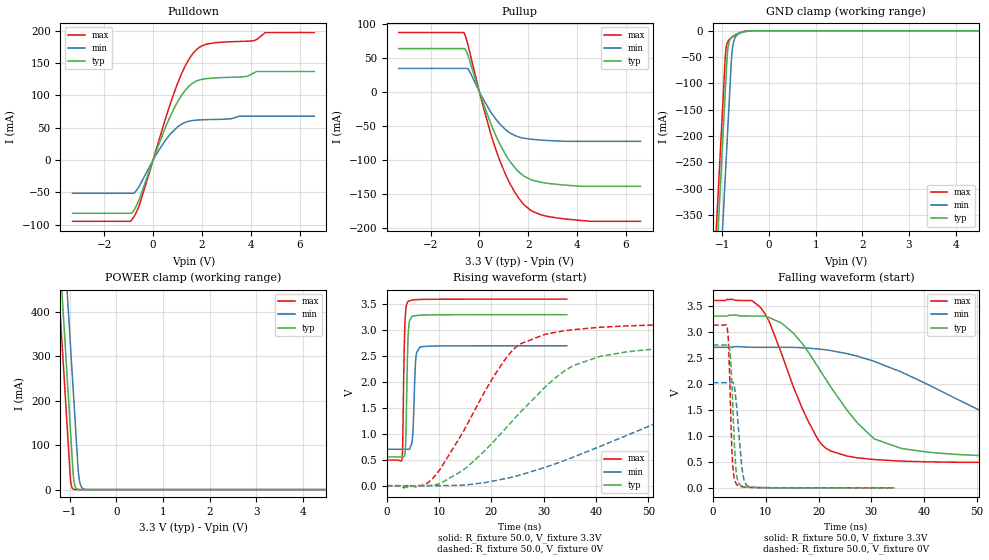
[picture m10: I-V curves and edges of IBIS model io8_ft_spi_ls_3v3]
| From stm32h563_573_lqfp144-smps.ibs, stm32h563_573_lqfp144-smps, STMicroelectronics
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[Model]   io8_ft_spi_ls_3v3
Model_type I/O
Polarity   Non-Inverting
Enable   Active-Low
| CAP_THRESHOLD on pad IOFT is "UDTCAPC" :
| Rising=20.0% of vddiom   Falling=80.0% of vddiom
| C_comp min and max val. don't necessarily correlate with the min and max pvt
| but are the smallest and greatest pad capacitance found.
| var   typ   min   max
C_comp   5.03667pF  4.97381pF  5.04450pF
|C_comp_pullup   3.26860pF  3.10795pF  3.04360pF
|C_comp_pulldown   1.76807pF  1.86586pF  2.00090pF
Vinl = 810.0mV
Vinh = 2.52V
Vmeas = 1.65V   | Reference voltage for timing measurements
Cref  = 50.0pF   | Timing specification test load capacitance value
Rref  = 100.0MOhm   | Timing specification test load resistance value
Vref  = 1.65V   | Timing specification test load voltage
[Model Spec]
| TIME_THRESHOLD on pin ZIV11 is "CMOS" :
| Rising=40.0% of vdd   Falling=60.0% of vdd
Vinl 1.29880V 1.07480V 1.40680V
Vinh 1.77520V 1.49320V 1.89720V
| variable   typ   min   max
[Temperature Range] 25.0 125.0 -40.0
| variable   typ   min   max
[Voltage Range] 3.3V 2.7V 3.6V
| variable   typ   min   max
[POWER Clamp Reference] 3.3V 2.7V 3.6V
| variable   typ   min   max
[GND Clamp Reference] 0V 0V 0V
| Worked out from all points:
|   slope of the pulldown table from 0 to 0.495 V, typ, clamps not added: 10 ohm
|   slope of the pullup table from 0 to 0.495 V, typ, clamps not added: 10 ohm
|   GND clamp passes 1 mA (typ) near -0.52 V on its own axis
|   POWER clamp passes 1 mA (typ) near -0.84 V on its own axis
|   rising waveform, R_fixture 50.0, V_fixture 3.3V: 20-80 % time 340ps typ, 425ps min, 327ps max; typ from 0.556 V to 3.3 V
|   falling waveform, R_fixture 50.0, V_fixture 3.3V: 20-80 % time 11.8ns typ, 26.7ns min, 7.44ns max; typ from 3.3 V to 0.556 V
|   rising waveform, R_fixture 50.0, V_fixture 0V: 20-80 % time 16.3ns typ, 32ns min, 11ns max; typ from 0 V to 2.74 V
|   falling waveform, R_fixture 50.0, V_fixture 0V: 20-80 % time 727ps typ, 1.05ns min, 588ps max; typ from 2.74 V to 0 V
[POWER Clamp]
-3.3V     4.068A     4.259A     3.957A
-1.25V    582.8mA    774.2mA    471.5mA
-1.13V    378.8mA    570.2mA    267.5mA
-1.09V    310.8mA    502.2mA    199.5mA
-1.02V    191.8mA    383.2mA    80.53mA
-990mV    140.8mA    332.2mA    29.53mA
-920mV    26.3mA     213.2mA    906uA
-880mV    5.543mA    145.2mA    123.7uA
-810mV    363.5uA    33.6mA     3.798uA
-770mV    76.62uA    10.47mA    519.4nA
-690mV    3.409uA    1.017mA    10.47nA
6.6V      0A         0A         0A
[GND Clamp]
-3.3V     -4.131A    -4.293A    -4.064A
-1.25V    -646.2mA   -808mA     -579.5mA
-940mV    -119.2mA   -281mA     -52.48mA
-920mV    -85.23mA   -247mA     -32.7mA
-900mV    -51.91mA   -213mA     -24.27mA
-870mV    -26.87mA   -162mA     -18.7mA
-810mV    -13.22mA   -60.41mA   -13.31mA
-790mV    -11.41mA   -38.37mA   -11.93mA
-740mV    -8.18mA    -15.37mA   -8.882mA
-660mV    -4.605mA   -6.274mA   -4.919mA
-320mV    -10.56uA   -77.76uA   -2.038uA
6.6V      9.514nA    1.879uA    704.5pA
| variable   typ   min   max
[Pullup Reference] 3.3V 2.7V 3.6V
| variable   typ   min   max
[Pulldown Reference] 0V 0V 0V
[Pullup]
-3.3V     63.89mA    34.71mA    87.52mA
-630mV    63.89mA    34.71mA    86.85mA
-430mV    49.62mA    32.06mA    63.53mA
120mV     -12.96mA   -8.365mA   -16.99mA
470mV     -47.29mA   -29.8mA    -62.21mA
800mV     -74.32mA   -45.73mA   -97.77mA
1.14V     -96.49mA   -57.59mA   -127.1mA
1.48V     -113mA     -64.78mA   -149.7mA
2.08V     -128.9mA   -69.61mA   -174.1mA
2.7V      -134.3mA   -71.45mA   -182.9mA
3.6V      -137.7mA   -72.9mA    -187.7mA
6.6V      -139.3mA   -72.9mA    -190.8mA
[Pulldown]
-3.3V     -82.43mA   -51.49mA   -94.82mA
-860mV    -81.66mA   -51.49mA   -91.78mA
-560mV    -60.16mA   -40.13mA   -69.41mA
120mV     12.61mA    7.999mA    15.37mA
800mV     75.3mA     43.94mA    97.52mA
1.33V     108.3mA    58.37mA    146.5mA
1.84V     123.1mA    61.83mA    172.7mA
2.51V     126.9mA    62.69mA    181.3mA
3.84V     129.3mA    67.77mA    183.7mA
4.13V     134.7mA    67.77mA    184.6mA
4.59V     136.9mA    67.77mA    197.1mA
6.6V      136.9mA    67.77mA    197.1mA
[Ramp]
dV/dt_r 1.64628V/16.22065ns 1.21218V/31.72839ns 1.87635V/10.80188ns
dV/dt_f 1.64665V/11.56808ns 1.19679V/26.48811ns 1.86387V/7.29972ns
R_load = 50.0
| Removed startup time: 0s 0s 0s  .
| Removed end time: 34.4ns.
[Rising Waveform]
R_fixture   = 50.0
V_fixture   = 3.3V
V_fixture_min = 2.7V
V_fixture_max = 3.6V
0s        555.6mV    703.3mV    493.6mV
2.9ns     555.7mV    703.3mV    509.6mV
3.05ns    553.1mV    703.3mV    815.2mV
3.4ns     581.7mV    703.4mV    2.898V
3.6ns     776.2mV    703.4mV    3.348V
4.1ns     2.914V     701mV      3.555V
4.85ns    3.266V     855.2mV    3.581V
5.55ns    3.282V     2.443V     3.589V
6.35ns    3.29V      2.676V     3.593V
34.4ns    3.3V       2.699V     3.6V
| Removed startup time: 0s 0s 0s  .
| Removed end time: 249.4ns.
[Falling Waveform]
R_fixture   = 50.0
V_fixture   = 3.3V
V_fixture_min = 2.7V
V_fixture_max = 3.6V
0s        3.3V       2.7V       3.6V
8.8ns     3.299V     2.7V       3.486V
15.25ns   2.97V      2.699V     1.934V
20.05ns   2.296V     2.667V     907.7mV
27.35ns   1.248V     2.53V      578mV
30.55ns   940.7mV    2.43V      543.7mV
40.75ns   685.5mV    1.984V     499.6mV
58.85ns   594.3mV    1.148V     488.3mV
76.35ns   570.4mV    888.9mV    490.3mV
249.4ns   555.6mV    705.3mV    493.6mV
| Removed startup time: 0s 0s 0s  .
| Removed end time: 249.4ns.
[Rising Waveform]
R_fixture   = 50.0
V_fixture   = 0V
V_fixture_min = 0V
V_fixture_max = 0V
0s        103.7nV    446.5nV    93.93nV
7.9ns     1.334mV    -337.5uV   59.97mV
14.5ns    293.5mV    10.02mV    1.02V
20.4ns    850.3mV    90.42mV    2.102V
24.6ns    1.316V     182.1mV    2.667V
35.6ns    2.315V     549.1mV    3.01V
45.8ns    2.581V     968.6mV    3.083V
61.1ns    2.69V      1.549V     3.114V
81.5ns    2.729V     1.872V     3.124V
249.4ns   2.744V     2.02V      3.127V
| Removed startup time: 0s 0s 0s  .
| Removed end time: 34.35ns.
[Falling Waveform]
R_fixture   = 50.0
V_fixture   = 0V
V_fixture_min = 0V
V_fixture_max = 0V
0s        2.744V     2.021V     3.127V
2.7ns     2.747V     2.021V     3.061V
2.95ns    2.742V     2.021V     2.734V
3.25ns    2.552V     2.021V     1.785V
3.7ns     1.715V     2.03V      476mV
4.2ns     555.7mV    1.83V      118.3mV
4.6ns     171.9mV    1.421V     54.6mV
5.7ns     26.13mV    235.3mV    19.13mV
7ns       11.98mV    19.05mV    9.014mV
34.35ns   205.6uV    372.5uV    149.6uV
